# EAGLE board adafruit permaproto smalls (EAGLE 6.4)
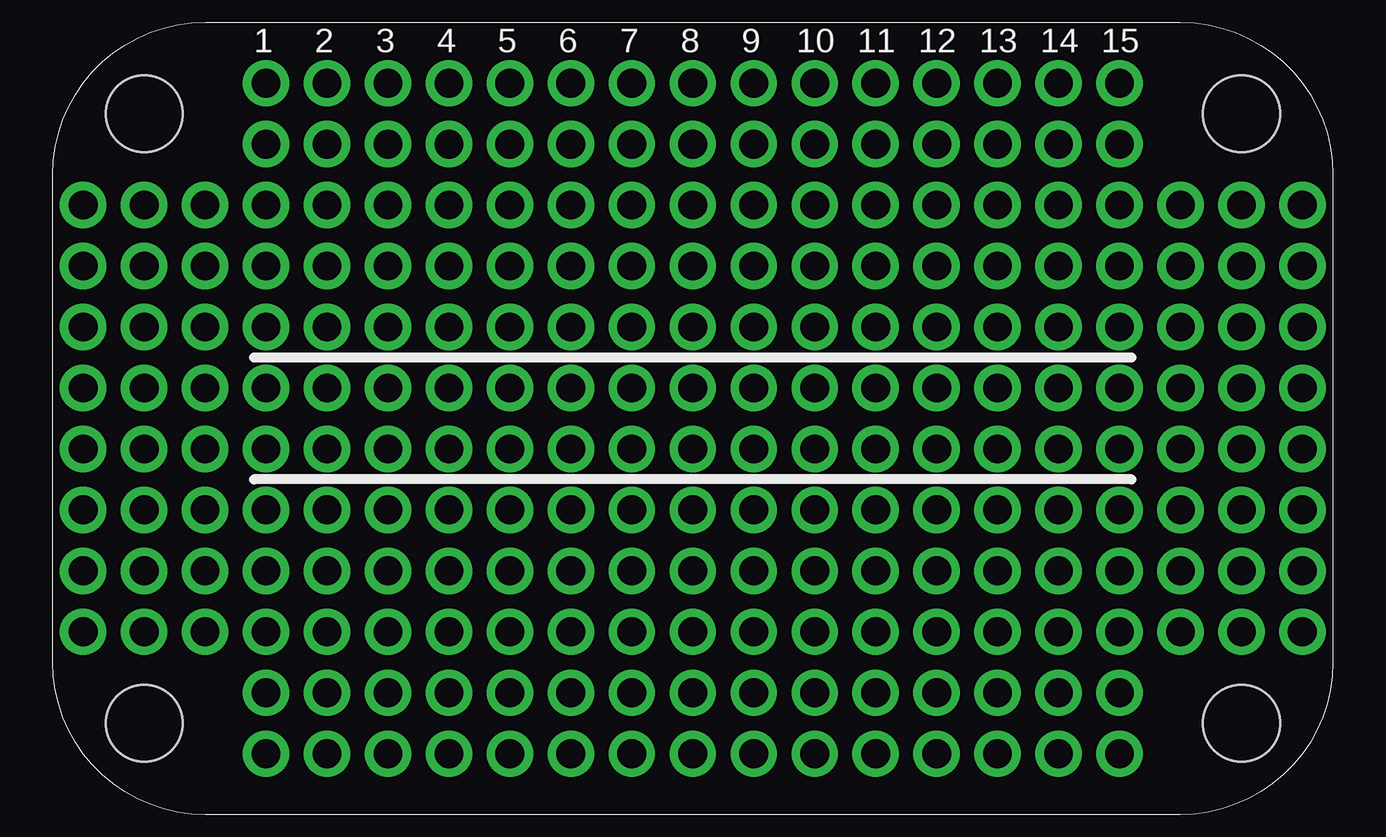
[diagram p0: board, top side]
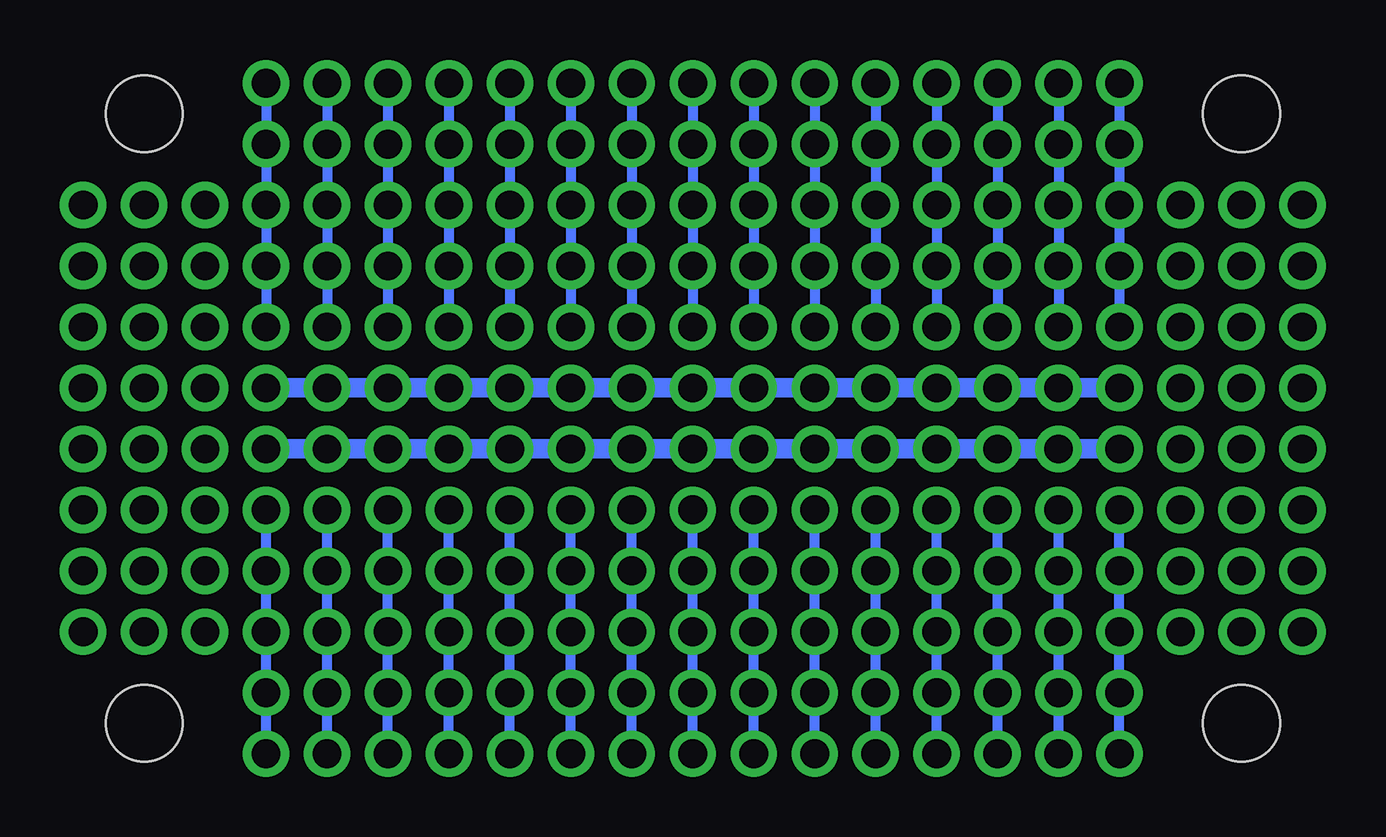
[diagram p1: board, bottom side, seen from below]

No outline drawn. Coordinates in mm, seen from the top.
Copper layers (1*16): Top 0.035mm / dielectric 1.5mm / Bottom 0.035mm
Design rules "default": minimum track width 10mil, minimum drill 24mil, track to track 8mil, track to pad 8mil, pad to pad 8mil, via to via 8mil, smd to smd 8mil, copper to edge 40mil, drill to drill 8mil, minimum pad ring 10mil, minimum via ring 8mil, stop-mask expansion 4mil, vias tented up to drill 0mil, thermal gap 10mil
Holes 3.2 mm at -22.86,12.7 22.86,12.7 -22.86,-12.7 22.86,-12.7

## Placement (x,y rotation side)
U$2  [ALTOIDSSMALLS]  0,0 90 top

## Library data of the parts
U$2 = adafruit

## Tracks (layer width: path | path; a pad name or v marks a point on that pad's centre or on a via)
A  (via drill 1.2 pad 1.93)
  Bottom 0.406: v-17.78,-3.81 v-17.78,-6.35 v-17.78,-8.89 v-17.78,-11.43 v-17.78,-13.97
AA  (via drill 1.2 pad 1.93)
  Bottom 0.406: v-10.16,13.97 v-10.16,11.43 v-10.16,8.89 v-10.16,6.35 v-10.16,3.81
B  (via drill 1.2 pad 1.93)
  Bottom 0.406: v-15.24,-13.97 v-15.24,-11.43 v-15.24,-8.89 v-15.24,-6.35 v-15.24,-3.81
BB  (via drill 1.2 pad 1.93)
  Bottom 0.406: v-12.7,3.81 v-12.7,6.35 v-12.7,8.89 v-12.7,11.43 v-12.7,13.97
C  (via drill 1.2 pad 1.93)
  Bottom 0.406: v-12.7,-3.81 v-12.7,-6.35 v-12.7,-8.89 v-12.7,-11.43 v-12.7,-13.97
CC  (via drill 1.2 pad 1.93)
  Bottom 0.406: v-15.24,3.81 v-15.24,6.35 v-15.24,8.89 v-15.24,11.43 v-15.24,13.97
D  (via drill 1.2 pad 1.93)
  Bottom 0.406: v-10.16,-13.97 v-10.16,-11.43 v-10.16,-8.89 v-10.16,-6.35 v-10.16,-3.81
DD  (via drill 1.2 pad 1.93)
  Bottom 0.406: v-17.78,13.97 v-17.78,11.43 v-17.78,8.89 v-17.78,6.35 v-17.78,3.81
E  (via drill 1.2 pad 1.93)
  Bottom 0.406: v-7.62,-3.81 v-7.62,-6.35 v-7.62,-8.89 v-7.62,-11.43 v-7.62,-13.97
F  (via drill 1.2 pad 1.93)
  Bottom 0.406: v-5.08,-13.97 v-5.08,-11.43 v-5.08,-8.89 v-5.08,-6.35 v-5.08,-3.81
G  (via drill 1.2 pad 1.93)
  Bottom 0.406: v-2.54,-3.81 v-2.54,-6.35 v-2.54,-8.89 v-2.54,-11.43 v-2.54,-13.97
GND  (via drill 1.2 pad 1.93)
  Bottom 0.813: v17.78,1.27 v15.24,1.27 v12.7,1.27 v10.16,1.27 v7.62,1.27 v5.08,1.27 v2.54,1.27 v0,1.27 v-2.54,1.27 v-5.08,1.27 v-7.62,1.27 v-10.16,1.27 v-12.7,1.27 v-15.24,1.27 v-17.78,1.27
H  (via drill 1.2 pad 1.93)
  Bottom 0.406: v0,-13.97 v0,-11.43 v0,-8.89 v0,-6.35 v0,-3.81
I  (via drill 1.2 pad 1.93)
  Bottom 0.406: v2.54,-3.81 v2.54,-6.35 v2.54,-8.89 v2.54,-11.43 v2.54,-13.97
J  (via drill 1.2 pad 1.93)
  Bottom 0.406: v5.08,-3.81 v5.08,-6.35 v5.08,-8.89 v5.08,-11.43 v5.08,-13.97
K  (via drill 1.2 pad 1.93)
  Bottom 0.406: v7.62,-3.81 v7.62,-6.35 v7.62,-8.89 v7.62,-11.43 v7.62,-13.97
L  (via drill 1.2 pad 1.93)
  Bottom 0.406: v10.16,-13.97 v10.16,-11.43 v10.16,-8.89 v10.16,-6.35 v10.16,-3.81
M  (via drill 1.2 pad 1.93)
  Bottom 0.406: v12.7,-3.81 v12.7,-6.35 v12.7,-8.89 v12.7,-11.43 v12.7,-13.97
N  (via drill 1.2 pad 1.93)
  Bottom 0.406: v15.24,-13.97 v15.24,-11.43 v15.24,-8.89 v15.24,-6.35 v15.24,-3.81
N$16  (via drill 1.2 pad 1.93)
  other vias: -20.32,8.89
N$17  (via drill 1.2 pad 1.93)
  other vias: -20.32,6.35
N$18  (via drill 1.2 pad 1.93)
  other vias: -20.32,3.81
N$19  (via drill 1.2 pad 1.93)
  other vias: -22.86,3.81
N$20  (via drill 1.2 pad 1.93)
  other vias: -22.86,6.35
N$21  (via drill 1.2 pad 1.93)
  other vias: -22.86,8.89
N$22  (via drill 1.2 pad 1.93)
  other vias: -25.4,8.89
N$23  (via drill 1.2 pad 1.93)
  other vias: -25.4,6.35
N$24  (via drill 1.2 pad 1.93)
  other vias: -25.4,3.81
N$25  (via drill 1.2 pad 1.93)
  other vias: -25.4,1.27
N$26  (via drill 1.2 pad 1.93)
  other vias: -22.86,1.27
N$27  (via drill 1.2 pad 1.93)
  other vias: -20.32,1.27
N$28  (via drill 1.2 pad 1.93)
  other vias: -20.32,-1.27
N$29  (via drill 1.2 pad 1.93)
  other vias: -22.86,-1.27
N$30  (via drill 1.2 pad 1.93)
  other vias: -25.4,-1.27
N$31  (via drill 1.2 pad 1.93)
  other vias: -25.4,-3.81
N$32  (via drill 1.2 pad 1.93)
  other vias: -22.86,-3.81
N$33  (via drill 1.2 pad 1.93)
  other vias: -20.32,-3.81
N$34  (via drill 1.2 pad 1.93)
  other vias: -20.32,-6.35
N$35  (via drill 1.2 pad 1.93)
  other vias: -22.86,-6.35
N$36  (via drill 1.2 pad 1.93)
  other vias: -25.4,-6.35
N$37  (via drill 1.2 pad 1.93)
  other vias: -25.4,-8.89
N$38  (via drill 1.2 pad 1.93)
  other vias: -22.86,-8.89
N$39  (via drill 1.2 pad 1.93)
  other vias: -20.32,-8.89
N$40  (via drill 1.2 pad 1.93)
  other vias: 20.32,8.89
N$41  (via drill 1.2 pad 1.93)
  other vias: 20.32,6.35
N$42  (via drill 1.2 pad 1.93)
  other vias: 20.32,3.81
N$43  (via drill 1.2 pad 1.93)
  other vias: 22.86,3.81
N$44  (via drill 1.2 pad 1.93)
  other vias: 22.86,6.35
N$45  (via drill 1.2 pad 1.93)
  other vias: 22.86,8.89
N$46  (via drill 1.2 pad 1.93)
  other vias: 25.4,8.89
N$47  (via drill 1.2 pad 1.93)
  other vias: 25.4,6.35
N$65  (via drill 1.2 pad 1.93)
  other vias: 25.4,3.81
N$66  (via drill 1.2 pad 1.93)
  other vias: 25.4,1.27
N$67  (via drill 1.2 pad 1.93)
  other vias: 25.4,-1.27
N$68  (via drill 1.2 pad 1.93)
  other vias: 25.4,-3.81
N$69  (via drill 1.2 pad 1.93)
  other vias: 25.4,-6.35
N$70  (via drill 1.2 pad 1.93)
  other vias: 25.4,-8.89
N$71  (via drill 1.2 pad 1.93)
  other vias: 22.86,-8.89
N$72  (via drill 1.2 pad 1.93)
  other vias: 20.32,-8.89
N$73  (via drill 1.2 pad 1.93)
  other vias: 22.86,-6.35
N$74  (via drill 1.2 pad 1.93)
  other vias: 20.32,-6.35
N$75  (via drill 1.2 pad 1.93)
  other vias: 20.32,-3.81
N$76  (via drill 1.2 pad 1.93)
  other vias: 22.86,-3.81
N$77  (via drill 1.2 pad 1.93)
  other vias: 22.86,-1.27
N$78  (via drill 1.2 pad 1.93)
  other vias: 20.32,-1.27
N$79  (via drill 1.2 pad 1.93)
  other vias: 20.32,1.27
N$80  (via drill 1.2 pad 1.93)
  other vias: 22.86,1.27
O  (via drill 1.2 pad 1.93)
  Bottom 0.406: v17.78,-13.97 v17.78,-11.43 v17.78,-8.89 | v17.78,-8.89 v17.78,-6.35 | v17.78,-6.35 v17.78,-3.81 | v17.78,-8.89 v17.78,-6.35
P  (via drill 1.2 pad 1.93)
  Bottom 0.406: v17.78,3.81 v17.78,6.35 v17.78,8.89 v17.78,11.43 v17.78,13.97
PWR  (via drill 1.2 pad 1.93)
  Bottom 0.813: v17.78,-1.27 v15.24,-1.27 v12.7,-1.27 v10.16,-1.27 v7.62,-1.27 v5.08,-1.27 v2.54,-1.27 v0,-1.27 v-2.54,-1.27 v-5.08,-1.27 v-7.62,-1.27 v-10.16,-1.27 v-12.7,-1.27 v-15.24,-1.27 v-17.78,-1.27
Q  (via drill 1.2 pad 1.93)
  Bottom 0.406: v15.24,13.97 v15.24,11.43 v15.24,8.89 v15.24,6.35 v15.24,3.81
R  (via drill 1.2 pad 1.93)
  Bottom 0.406: v12.7,3.81 v12.7,6.35 v12.7,8.89 v12.7,11.43 v12.7,13.97
S  (via drill 1.2 pad 1.93)
  Bottom 0.406: v10.16,3.81 v10.16,6.35 v10.16,8.89 v10.16,11.43 v10.16,13.97
T  (via drill 1.2 pad 1.93)
  Bottom 0.406: v7.62,13.97 v7.62,11.43 v7.62,8.89 v7.62,6.35 v7.62,3.81
U  (via drill 1.2 pad 1.93)
  Bottom 0.406: v5.08,3.81 v5.08,6.35 v5.08,8.89 v5.08,11.43 v5.08,13.97
V  (via drill 1.2 pad 1.93)
  Bottom 0.406: v2.54,13.97 v2.54,11.43 v2.54,8.89 v2.54,6.35 v2.54,3.81
W  (via drill 1.2 pad 1.93)
  Bottom 0.406: v0,3.81 v0,6.35 v0,8.89 v0,11.43 v0,13.97
X  (via drill 1.2 pad 1.93)
  Bottom 0.406: v-2.54,13.97 v-2.54,11.43 v-2.54,8.89 v-2.54,6.35 v-2.54,3.81
Y  (via drill 1.2 pad 1.93)
  Bottom 0.406: v-5.08,3.81 v-5.08,6.35 v-5.08,8.89 v-5.08,11.43 v-5.08,13.97
Z  (via drill 1.2 pad 1.93)
  Bottom 0.406: v-7.62,13.97 v-7.62,11.43 v-7.62,8.89 v-7.62,6.35 v-7.62,3.81

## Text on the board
tPlace: 1 | 2 | 3 | 4 | 5 | 6 | 7 | 8 | 9 | 10 | 11 | 12 | 13 | 14 | 15
tDocu: Adafruit Perma-Proto Small Tin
